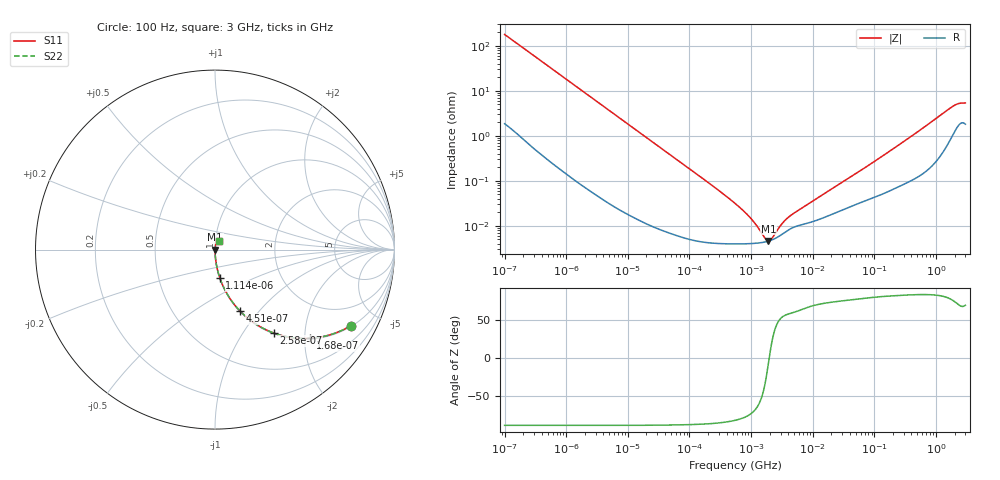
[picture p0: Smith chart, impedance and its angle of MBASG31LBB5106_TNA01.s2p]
! MBASG31LBB5106_TNA01  S-PARAMETER MODEL  ( Standard Model )
! Model Generated by TAIYO YUDEN Corporation (http://www.ty-top.com)
! Version 1.0
! TAIYO YUDEN Control No. 220601
! Copyright(c) 2015 TAIYO YUDEN CO.,LTD. All Rights Reserved.
! Product Description (link to TY-COMPAS)
! https://ds.yuden.co.jp/TYCOMPAS/or/detail?pn=MBASG31LBB5106KTNA01&u=M
! Products Name : Multilayer Ceramic Capacitors
! Characteristics :
!  Capacitance : 10 [uF] , Rated Voltage : 35 [V] , TCC : X5R
!  Case Size : 3.2 x 1.6 / 0.126 x 0.063 [mm/inch] , Thickness : 1.6 / 0.063 [mm/inch]
!  (Conditions: Temperature = 25 [degC] , DC Bias Voltage = 0 [V])
! External Node Assignments :
!  1  o---| |---o  2
! GND o---------o GND
! Frequency Range : 100Hz  -  3GHz  [ 401 STEP ]
# MHZ S RI R 50
! Freq[MHz].  S11 Real  S11 Imag  S21 Real  S21 Imag  S12 Real  S12 Imag  S22 Real  S22 Imag
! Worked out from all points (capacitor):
!   401 points, 100 Hz to 3 GHz, reference 50 ohm
!   read as one part in series: C = 8.94 uF near 109 Hz
!   lowest |Z| = 4.57 mohm at 1.908 MHz (marker M1)
!   series resonance near 1.966 MHz, so ESL is about 730 pH
!   S11 on the Smith chart (normalised r, x): 100 Hz: 1.04, -3.55; 168 Hz: 1.02, -2.13; 258 Hz: 1.01, -1.39; 451 Hz: 1.01, -0.80; 1.114 kHz: 1.00, -0.32; 3 GHz: 1.04, +0.10
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0.0001  0.7572 -0.4236  0.2428 0.4236  0.2428 0.4236  0.7572 -0.4236
0.000168  0.5309 -0.4942  0.4691 0.4942  0.4691 0.4942  0.5309 -0.4942
0.000258  0.3265 -0.4645  0.6735 0.4645  0.6735 0.4645  0.3265 -0.4645
0.000451  0.1386 -0.3414  0.8614 0.3414  0.8614 0.3414  0.1386 -0.3414
0.000664  0.0699 -0.251  0.9301 0.251  0.9301 0.251  0.0699 -0.251
0.001114  0.0267 -0.1572  0.9733 0.1572  0.9733 0.1572  0.0267 -0.1572
0.001788  0.0108 -0.0998  0.9892 0.0998  0.9892 0.0998  0.0108 -0.0998
0.005476  0.00138 -0.0331  0.9986 0.0331  0.9986 0.0331  0.00138 -0.0331
0.031977  0.000116 -0.00572  0.9999 0.00572  0.9999 0.00572  0.000116 -0.00572
0.221826  4.19e-05 -0.000822  1 0.000822  1 0.000822  4.19e-05 -0.000822
0.547723  3.94e-05 -0.000312  1 0.000312  1 0.000312  3.94e-05 -0.000312
0.806856  3.96e-05 -0.000191  1 0.000191  1 0.000191  3.96e-05 -0.000191
1.240863  4.09e-05 -9.01e-05  1 9.01e-05  1 9.01e-05  4.09e-05 -9.01e-05
1.352413  4.14e-05 -7.25e-05  1 7.25e-05  1 7.25e-05  4.14e-05 -7.25e-05
1.908323  4.54e-05 -5.59e-06  1 5.59e-06  1 5.59e-06  4.54e-05 -5.59e-06
2.93481  6e-05 7.56e-05  0.9999 -7.56e-05  0.9999 -7.56e-05  6e-05 7.56e-05
4.513443  8.75e-05 0.00015  0.9999 -0.00015  0.9999 -0.00015  8.75e-05 0.00015
9.794414  0.000122 0.000323  0.9999 -0.000323  0.9999 -0.000323  0.000122 0.000323
175.1444  0.000608 0.00444  0.9994 -0.00444  0.9994 -0.00444  0.000608 0.00444
1789.813  0.0108 0.0413  0.9892 -0.0413  0.9892 -0.0413  0.0108 0.0413
2317.205  0.0188 0.0473  0.9812 -0.0473  0.9812 -0.0473  0.0188 0.0473
3000  0.0201 0.0484  0.9799 -0.0484  0.9799 -0.0484  0.0201 0.0484
